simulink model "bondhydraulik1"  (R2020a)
settings: Solver=ode45  StartTime=0.0  StopTime=2  RelTol=1e-3  EnableMultiTasking=on
undefined symbols (not defined in the file or in its folder): Display, Int, libbondgraph
libraries: libbondgraph x5

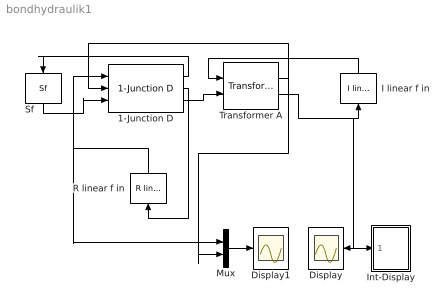
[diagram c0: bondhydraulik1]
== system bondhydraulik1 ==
  1-Junction D : libbondgraph/1-Junction D
  Display : Scope
  Display1 : Scope
  I linear f in : libbondgraph/I linear f in  I=500
  Int-Display : Subsystem  AncestorBlock=libbondgraph/Int-Display
  Mux : Mux  Inputs=2
  R linear f in : libbondgraph/R linear f in  R=8e7
  Sf : libbondgraph/Sf  f_ext=0.001
  Transformer A : libbondgraph/Transformer A  m=1000
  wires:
  Mux/1 -> Display1/1
  Sf/1 -> 1-Junction D/3
  1-Junction D/1 -> Sf/1
  1-Junction D/2 -> R linear f in/1
  R linear f in/1 -> 1-Junction D/1, Mux/1
  1-Junction D/3 -> Transformer A/2
  Transformer A/1 -> 1-Junction D/2, Mux/2
  Transformer A/2 -> I linear f in/1, Display/1, Int-Display/1(In1)
  I linear f in/1 -> Transformer A/1

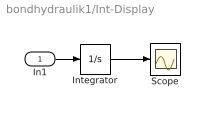
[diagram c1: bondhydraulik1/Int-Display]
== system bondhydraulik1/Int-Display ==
  In1 : Inport
  Integrator : Integrator
  Scope : Scope
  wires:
  In1/1 -> Integrator/1
  Integrator/1 -> Scope/1
